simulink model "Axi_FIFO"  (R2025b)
settings: Solver=VariableStepAuto  StartTime=0.0  StopTime=100  RelTol=1e-3
undefined symbols (not defined in the file or in its folder): AXI_FIFO_config, sysgen
libraries: hdlUtilities x2, simulink x1, hdlBasic x1, dspsrcs4 x1

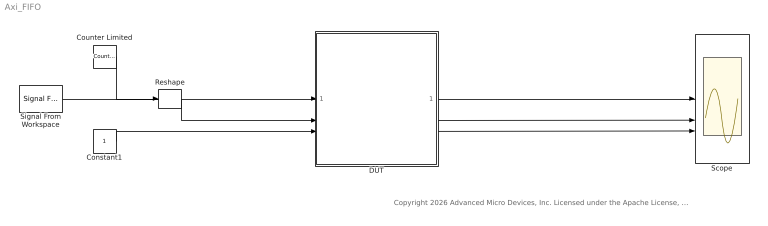
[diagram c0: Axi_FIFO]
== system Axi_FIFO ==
  note: Copyright 2026 Advanced Micro Devices, Inc. Licensed under the Apache License, Version 2.0 (the "License"); you may not use this file except in compliance with the License. You may obtain a copy of the License at http://www.apache.org/licenses/LICENSE-2.0 Unless required by applicable law or agreed to in writing, software distributed under the License is distributed on an "AS IS" BASIS, WITHOUT WARRANTIES OR CONDITIONS OF ANY KIND, either express or implied. See the License for the specific language governing permissions and limitations under the License.
  Constant1 : Constant  OutDataTypeStr=boolean  SampleTime=-1
  Counter Limited : simulink/Sources/Counter Limited  uplimit=7  tsamp=1
  DUT : Subsystem
  Reshape : Reshape  OutputDimensionality=Customize  OutputDimensions=[1]
  Scope : Scope  NumInputPorts=3
  Signal From Workspace : dspsrcs4/Signal From Workspace  X=[1 1 0 0 1 1 1 0]  Ts=-1  nsamps=1  OutputAfterFinalValue=Cyclic repetition  ignoreOrWarnInputAndFrameLengths=off  OutputFrames=off
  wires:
  Counter Limited/1 -> DUT/1(data_in)
  Signal From Workspace/1 -> Reshape/1
  Constant1/1 -> DUT/3(ready_in)
  DUT/1(data_out) -> Scope/1
  DUT/2(valid_out) -> Scope/2
  DUT/3(ready_out) -> Scope/3
  Reshape/1 -> DUT/2(valid_in)

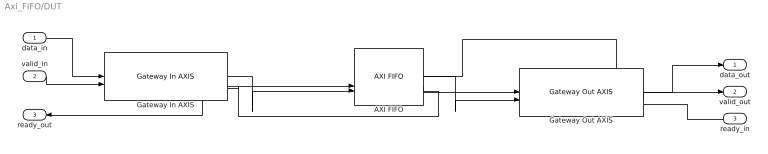
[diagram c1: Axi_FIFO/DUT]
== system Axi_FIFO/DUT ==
  data_in : Inport
  valid_in : Inport  Port=2
  ready_in : Inport  Port=3
  AXI FIFO : hdlBasic/AXI FIFO  input_depth_axis=1K  actual_fifo_depth_label=1026  enable_tdata=on  enable_tdest=off  enable_tstrb=off  enable_tready=on  enable_tid=off  enable_tuser=off  enable_tkeep=off  enable_tlast=off  has_aresetn=off  enable_data_counts_axis=off  fifo_implementation_type_axis=Common Clock Block RAM  trim_axipin_name=on  programmable_full_type_axis=Full  full_threshold_assert_value_axis=0  programmable_empty_type_axis=Empty  empty_threshold_assert_value_axis=1022  underflow_flag_axi=0  underflow_sense_axi=Active High  overflow_flag_axi=0  overflow_sense_axi=Active High  simulation_type=fast_sim  XmcBlockStatus=1  maskContainerNames=tabcontainer1  block_type=axi_fifo  block_config=sysgen:AXI_FIFO_config
  Gateway In AXIS : hdlUtilities/Gateway In AXIS  gui_display_data_type=Fixed-point  arith_type=Signed (2's comp)  n_bits=32  bin_pt=0  preci_type=Custom  exp_width=16  frac_width=24  quantization=Truncate  overflow=Flag as error  OutSampleTime=1  block_type=gatewayinaxi  XmcBlockStatus=1
  Gateway Out AXIS : hdlUtilities/Gateway Out AXIS  mask_sample_period=1  block_type=gatewayoutaxi
  data_out : Outport
  valid_out : Outport  Port=2
  ready_out : Outport  Port=3
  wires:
  AXI FIFO/3 -> Gateway In AXIS/3
  data_in/1 -> Gateway In AXIS/1
  Gateway In AXIS/1 -> AXI FIFO/3
  Gateway In AXIS/2 -> AXI FIFO/2
  valid_in/1 -> Gateway In AXIS/2
  Gateway In AXIS/3 -> ready_out/1
  AXI FIFO/1 -> Gateway Out AXIS/2
  AXI FIFO/2 -> Gateway Out AXIS/1
  Gateway Out AXIS/2 -> valid_out/1
  ready_in/1 -> Gateway Out AXIS/3
  Gateway Out AXIS/1 -> data_out/1
  Gateway Out AXIS/3 -> AXI FIFO/1
